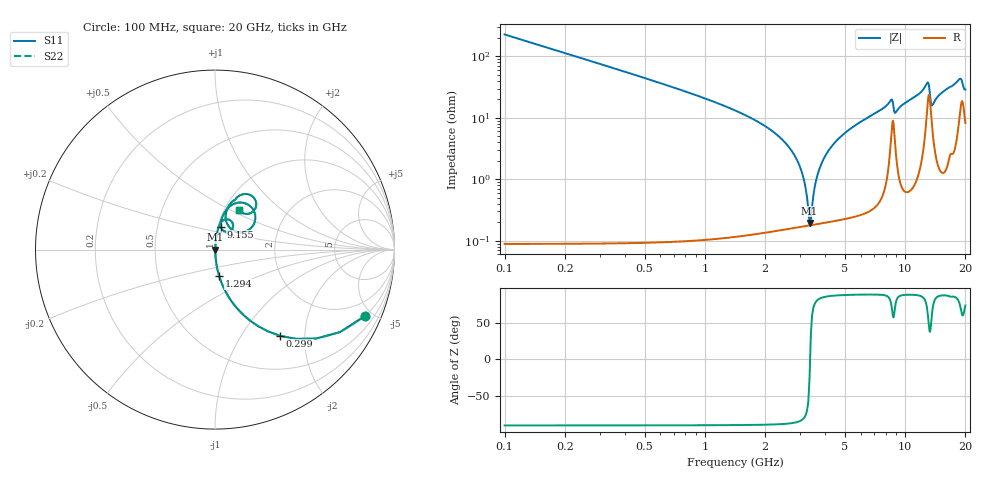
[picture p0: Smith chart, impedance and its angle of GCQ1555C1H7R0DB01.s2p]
!Murata Part Number: GCQ1555C1H7R0DB01
!These Parameters are Measured in Series Mode Connection
!Data Generated on Jan 08, 2026
!  o--ll--o
!Port1  Port2
!  o------o
!Operation Temp=25[degC], DC Bias Voltage=0[V]
!Freq. Start=100[MHz] Stop=20[GHz] 401[Steps]
# Hz S RI R 50
!Freq.(Hz) S11(Real) S11(Imag) S21(Real) S21(Imag) S12(Real) S12(Imag) S22(Real) S22(Imag)
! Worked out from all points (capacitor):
!   401 points, 100 MHz to 20 GHz, reference 50 ohm
!   read as one part in series: C = 7 pF near 199.5 MHz
!   lowest |Z| = 195 mohm at 3.334 GHz (marker M1)
!   series resonance near 3.354 GHz, so ESL is about 320 pH
!   S11 on the Smith chart (normalised r, x): 100 MHz: 1.00, -4.54; 299 MHz: 1.00, -1.51; 1.294 GHz: 1.00, -0.30; 9.155 GHz: 1.03, +0.27; 20 GHz: 1.16, +0.55
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1e8  0.8376 -0.3686  0.1624 0.3686  0.1624 0.3686  0.8376 -0.3686
2.99e8  0.3628 -0.4802  0.6372 0.4802  0.6372 0.4802  0.3628 -0.4802
5.975e8  0.1201 -0.3238  0.8799 0.3238  0.8799 0.3238  0.1201 -0.3238
1.294e9  0.0229 -0.1459  0.9771 0.1459  0.9771 0.1459  0.0229 -0.1459
2.73675e9  0.00236 -0.0277  0.9976 0.0277  0.9976 0.0277  0.00236 -0.0277
3.03525e9  0.00187 -0.0135  0.9981 0.0135  0.9981 0.0135  0.00187 -0.0135
3.33375e9  0.00177 -0.0008  0.9982 0.0008  0.9982 0.0008  0.00177 -0.0008
3.43325e9  0.00181 0.00319  0.9982 -0.00319  0.9982 -0.00319  0.00181 0.00319
3.73175e9  0.0021 0.0145  0.9979 -0.0145  0.9979 -0.0145  0.0021 0.0145
4.22925e9  0.00304 0.0318  0.997 -0.0318  0.997 -0.0318  0.00304 0.0318
5.1745e9  0.00607 0.0612  0.9939 -0.0612  0.9939 -0.0612  0.00607 0.0612
6.7665e9  0.0146 0.1066  0.9854 -0.1066  0.9854 -0.1066  0.0146 0.1066
8.50775e9  0.0747 0.1679  0.9253 -0.1679  0.9253 -0.1679  0.0747 0.1679
8.856e9  0.0584 0.1003  0.9416 -0.1003  0.9416 -0.1003  0.0584 0.1003
9.1545e9  0.0318 0.1273  0.9682 -0.1273  0.9682 -0.1273  0.0318 0.1273
1.005e10  0.0358 0.169  0.9642 -0.169  0.9642 -0.169  0.0358 0.169
1.288575e10  0.1929 0.2448  0.8071 -0.2448  0.8071 -0.2448  0.1929 0.2448
1.338325e10  0.1429 0.0961  0.8571 -0.0961  0.8571 -0.0961  0.1429 0.0961
1.3632e10  0.0837 0.1209  0.9163 -0.1209  0.9163 -0.1209  0.0837 0.1209
1.67165e10  0.1079 0.2747  0.8921 -0.2747  0.8921 -0.2747  0.1079 0.2747
1.875625e10  0.2116 0.2939  0.7884 -0.2939  0.7884 -0.2939  0.2116 0.2939
2e10  0.1327 0.2215  0.8673 -0.2215  0.8673 -0.2215  0.1327 0.2215
